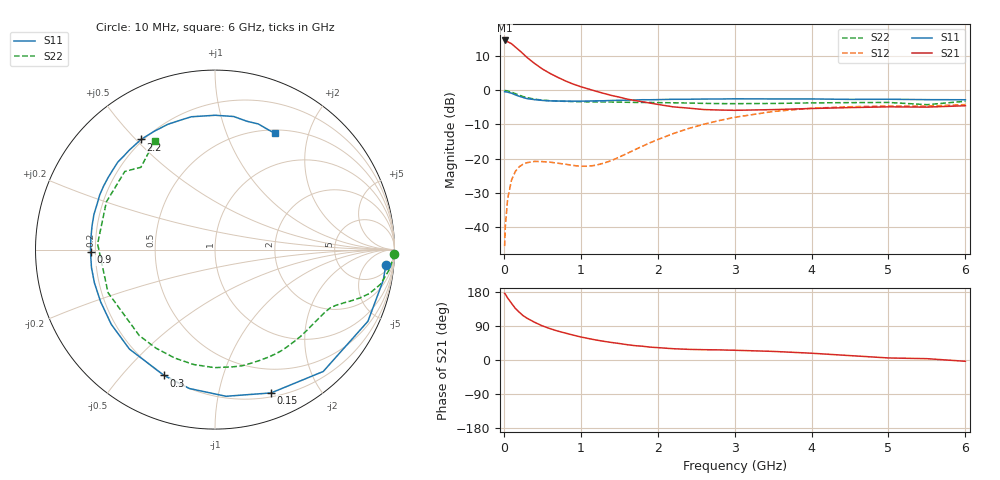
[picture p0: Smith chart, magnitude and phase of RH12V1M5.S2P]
! SIEMENS Small Signal Semiconductors
! BFR106
! Si NPN RF Bipolar Junction Transistor in SOT23
! VCE = 12 V  IC = 1.5 mA
! Common Emitter S-Parameters:  August  1996
# GHz  S  MA  R  50
!  f  S11  S21  S12  S22
! GHz  MAG  ANG  MAG  ANG  MAG  ANG  MAG  ANG
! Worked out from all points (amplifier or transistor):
!   36 points, 10 MHz to 6 GHz, reference 50 ohm
!   highest |S21| = 14.6 dB at 10 MHz (marker M1)
!   |S21| within 3 dB of that: start of sweep to 205.7 MHz
!   unconditionally stable (mu >= 1): 821.8 MHz to 1.794 GHz; 3.879 GHz to end of sweep
!   at 250 MHz: K = 0.29, MSG = 16.2 dB, |S12| = -21.6 dB
!   at 1.4 GHz: K = 1.28, MAG = 6.3 dB, |S12| = -20.6 dB
!   at 6 GHz: K = 1.02, MAG = -1.0 dB, |S12| = -4.2 dB
!   S11 on the Smith chart (normalised r, x): 10 MHz: 9, -18; 150 MHz: 0.24, -1.44; 300 MHz: 0.20, -0.66; 900 MHz: 0.18, -0.01; 2.2 GHz: 0.19, +0.52; 6 GHz: 0.54, +1.50
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0.01  0.9559 -5.1  5.388 176.0  0.0052 86.2  0.9999 -1.4
0.02  0.953 -10.3  5.338 173.6  0.0104 85.0  0.9943 -2.6
0.05  0.941 -25.1  5.163 163.4  0.0259 76.2  0.9797 -6.3
0.1  0.9081 -48.4  4.826 149.6  0.0485 64.6  0.9426 -11.8
0.15  0.8575 -68.6  4.308 136.0  0.065 53.6  0.8942 -15.9
0.2  0.8195 -85.7  3.866 126.3  0.0759 45.9  0.8502 -18.5
0.25  0.787 -100.4  3.438 117.1  0.0829 39.5  0.8108 -20.6
0.3  0.7563 -112.0  3.043 110.4  0.087 35.3  0.7829 -22.1
0.4  0.7311 -130.7  2.476 99.5  0.091 29.1  0.7433 -24.6
0.5  0.7124 -144.2  2.06 90.1  0.0903 25.7  0.7188 -26.9
0.7  0.697 -164.5  1.554 76.4  0.0856 25.3  0.6966 -32.4
0.9  0.6937 -178.8  1.237 65.8  0.0794 31.3  0.6847 -38.3
1.1  0.6978 169.0  1.047 56.7  0.0772 43.9  0.6791 -45.2
1.6  0.7181 146.1  0.745 40.5  0.1186 73.3  0.6686 -63.9
2.2  0.7394 123.9  0.573 29.8  0.2319 75.7  0.6577 -90.2
2.8  0.7463 105.3  0.515 26.7  0.3608 63.6  0.64 -121.1
3.5  0.7484 89.9  0.522 22.7  0.4901 45.8  0.6424 -158.0
4  0.7489 82.0  0.542 17.9  0.5469 33.1  0.6548 177.2
4.5  0.7368 76.1  0.559 11.6  0.575 21.9  0.6609 156.3
5  0.7404 71.0  0.573 5.4  0.5888 12.7  0.6649 139.1
5.5  0.7307 66.0  0.568 3.5  0.5872 8.2  0.617 132.0
6  0.7283 62.9  0.595 -3.4  0.6184 -0.2  0.6919 119.1
